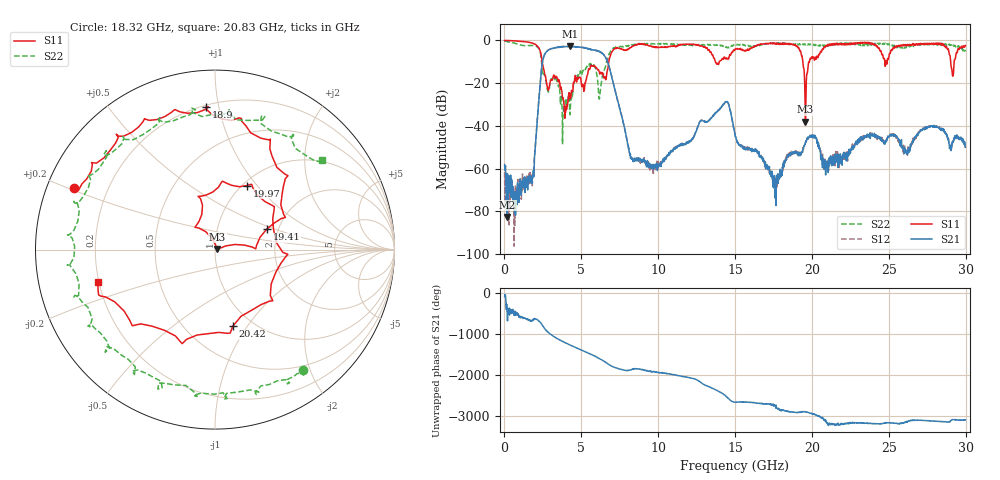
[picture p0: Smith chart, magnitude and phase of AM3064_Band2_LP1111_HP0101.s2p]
# Hz S DB R 50.0
!freq dBS11 angS11 dBS21 angS21 dBS12 angS12 dBS22 angS22
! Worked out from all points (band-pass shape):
!   1600 points, 10 MHz to 29.98 GHz, reference 50 ohm
!   highest |S21| = -2.78 dB at 4.246 GHz (marker M1); lowest = -82.6 dB at 178.7 MHz (marker M2)
!   |S21| within 3 dB of the highest: 2.682 GHz to 6.305 GHz (3.623 GHz wide, 80.6 % of centre)
!   lowest |S11| = -38.0 dB at 19.58 GHz (marker M3), VSWR 1.03, Z = 51.2 + j0.319 ohm
!   |S11| at or under -10 dB: 2.449 GHz to 6.786 GHz (4.336 GHz wide, 93.9 % of centre); 19.41 GHz to 19.83 GHz (427.1 MHz wide, 2.18 % of centre); 29.03 GHz to 29.25 GHz (227.5 MHz wide, 0.781 % of centre)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
!   |S22| runs from -48.6 to -0.1 dB; largest |S21 - S12| = 0.018
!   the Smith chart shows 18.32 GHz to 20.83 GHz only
!   S11 on the Smith chart (normalised r, x): 18.32 GHz: 0.08, +0.21; 18.9 GHz: 0.21, +0.92; 19.41 GHz: 1.74, +0.44; 19.97 GHz: 1.05, +0.89; 20.42 GHz: 0.81, -0.86; 20.83 GHz: 0.20, -0.13
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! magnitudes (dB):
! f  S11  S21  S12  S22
! 10 MHz  -0.1  -58.1  -61.7  -0.1
! 178.7 MHz  -0.1  -82.6  -65.6  -0.6
! 1.753 GHz  -1.2  -64.8  -65.9  -2.4
! 2.578 GHz  -14.2  -7.1  -7.2  -15.7
! 4.246 GHz  -24.9  -2.8  -2.8  -33.8
! 5.015 GHz  -20.7  -3.2  -3.2  -15.9
! 6.627 GHz  -17.2  -8.7  -8.6  -10.2
! 8.276 GHz  -2.9  -55.5  -55.1  -2.1
! 10 GHz  -3.3  -58.6  -58.8  -1.6
! 14.37 GHz  -8.6  -28.8  -28.7  -3.1
! 15 GHz  -4.1  -44.4  -44.4  -2.2
! 17.59 GHz  -1.2  -67.9  -65.7  -1.1
! 18.32 GHz  -1.3  -56.0  -55.6  -1.6
! 18.9 GHz  -2.0  -52.1  -52.6  -2.0
! 19.41 GHz  -10.2  -51.2  -50.2  -1.7
! 19.58 GHz  -38.0  -47.7  -47.9  -2.1
! 19.97 GHz  -8.0  -45.1  -44.7  -2.0
! 19.99 GHz  -7.7  -44.6  -44.7  -1.7
! 20.42 GHz  -7.2  -48.0  -49.8  -2.5
! 20.83 GHz  -3.4  -56.2  -58.2  -2.2
! 25 GHz  -8.1  -45.3  -44.9  -1.6
! 29.98 GHz  -2.4  -50.0  -50.5  -4.4
